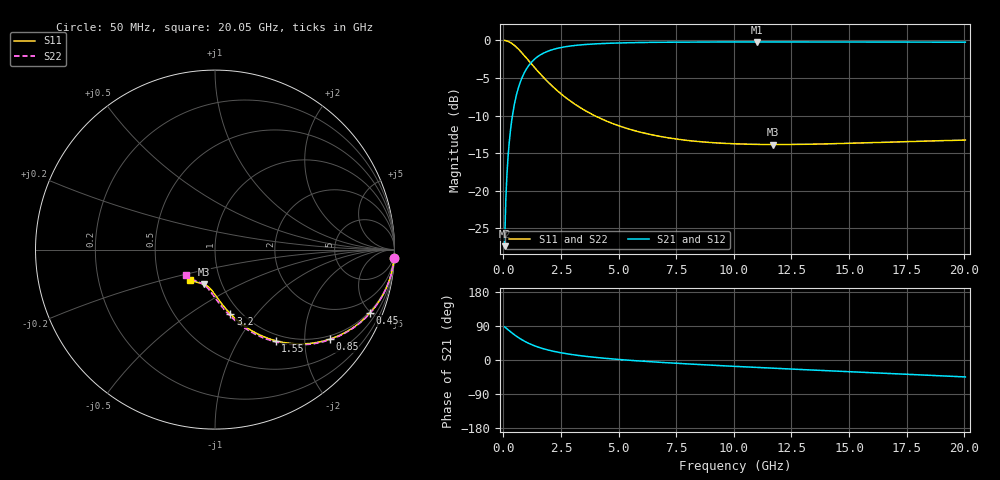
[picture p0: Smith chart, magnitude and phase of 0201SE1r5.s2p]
! AVX Thin Film Operation		Date: August 2001
! Description: Accu-P® Series, Thin Film, SMD, RF Capacitor
! Part Number: 02013J1R5ABW
! 50 MHz  -  20.05 GHz
! Serial Measurements
# mhz S db R 50
!	S11		S21		S12		S22
!	dB	Phase	dB	Phase	dB	Phase	dB	Phase
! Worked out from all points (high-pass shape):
!   401 points, 50 MHz to 20.05 GHz, reference 50 ohm
!   highest |S21| = -0.20 dB at 11 GHz (marker M1); lowest = -27.4 dB at 50 MHz (marker M2)
!   |S21| within 3 dB of the highest: 1.133 GHz to end of sweep
!   lowest |S11| = -13.9 dB at 11.7 GHz (marker M3), VSWR 1.51, Z = 41 - j16.5 ohm
!   |S11| at or under -10 dB: 3.949 GHz to end of sweep
!   |S22| runs from -13.9 to 0.0 dB; largest |S21 - S12| = 0
!   S11 on the Smith chart (normalised r, x): 50 MHz: 1, -44; 450 MHz: 0.90, -4.94; 850 MHz: 0.90, -2.63; 1.55 GHz: 0.90, -1.46; 3.2 GHz: 0.90, -0.74; 20.05 GHz: 0.72, -0.25
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50  -0.01 -2.6  -27.39 87.4  -27.39 87.4  -0.01 -2.6
100  -0.03 -5.1  -21.39 84.8  -21.39 84.8  -0.03 -5.2
200  -0.13 -10.2  -15.47 79.7  -15.47 79.7  -0.13 -10.3
250  -0.20 -12.7  -13.60 77.2  -13.60 77.2  -0.20 -12.8
350  -0.37 -17.6  -10.86 72.3  -10.86 72.3  -0.37 -17.7
450  -0.60 -22.2  -8.91 67.7  -8.91 67.7  -0.60 -22.4
650  -1.17 -30.7  -6.29 59.1  -6.29 59.1  -1.16 -31.0
850  -1.83 -38.0  -4.65 51.7  -4.65 51.7  -1.83 -38.5
1150  -2.90 -47.2  -3.13 42.5  -3.13 42.5  -2.90 -47.8
1550  -4.30 -56.4  -2.02 33.1  -2.02 33.1  -4.30 -57.2
1900  -5.44 -62.5  -1.47 26.9  -1.47 26.9  -5.44 -63.5
2250  -6.46 -67.3  -1.12 22.0  -1.12 22.0  -6.46 -68.5
3200  -8.69 -76.5  -0.64 12.5  -0.64 12.5  -8.69 -78.3
3400  -9.07 -78.0  -0.58 10.9  -0.58 10.9  -9.08 -79.8
4950  -11.30 -86.8  -0.35 1.7  -0.35 1.7  -11.31 -89.4
6750  -12.75 -93.8  -0.25 -5.9  -0.25 -5.9  -12.77 -97.3
10050  -13.76 -103.8  -0.20 -16.8  -0.20 -16.8  -13.79 -108.8
11000  -13.84 -106.4  -0.20 -19.6  -0.20 -19.6  -13.87 -111.8
11700  -13.86 -108.2  -0.20 -21.7  -0.20 -21.7  -13.89 -113.9
13400  -13.81 -112.6  -0.20 -26.5  -0.20 -26.5  -13.85 -119.1
16750  -13.54 -121.1  -0.22 -35.7  -0.22 -35.7  -13.60 -129.0
20050  -13.27 -129.3  -0.24 -44.7  -0.24 -44.7  -13.33 -138.7
